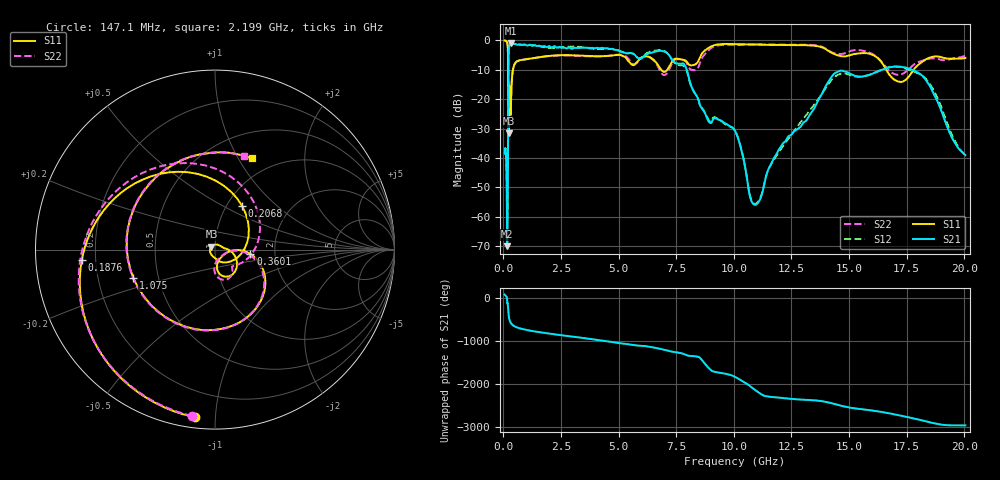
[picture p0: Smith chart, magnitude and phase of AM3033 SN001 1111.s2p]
# Hz S DB R 50
!freq MagS11 AngS11 MagS21 AngS21 MagS12 AngS12 MagS22 AngS22
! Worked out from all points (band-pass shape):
!   1601 points, 50 MHz to 20.05 GHz, reference 50 ohm
!   highest |S21| = -0.93 dB at 335.3 MHz (marker M1); lowest = -69.9 dB at 162.1 MHz (marker M2)
!   |S21| within 3 dB of the highest: 226.9 MHz to 5.122 GHz (4.895 GHz wide, 183 % of centre); 6.555 GHz to 7.022 GHz (466.9 MHz wide, 6.88 % of centre)
!   lowest |S11| = -31.6 dB at 225.4 MHz (marker M3), VSWR 1.05, Z = 48 + j1.65 ohm
!   |S11| at or under -10 dB: 205.8 MHz to 413.2 MHz (207.4 MHz wide, 67 % of centre); 6.839 GHz to 7.113 GHz (273.3 MHz wide, 3.92 % of centre); 16.61 GHz to 17.81 GHz (1.195 GHz wide, 6.94 % of centre)
!   |S22| runs from -25.9 to -0.1 dB; largest |S21 - S12| = 0.064
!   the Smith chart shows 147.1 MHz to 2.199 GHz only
!   S11 on the Smith chart (normalised r, x): 147.1 MHz: 0.05, -0.89; 187.6 MHz: 0.15, -0.04; 206.8 MHz: 1.18, +0.62; 360.1 MHz: 1.49, -0.08; 1.075 GHz: 0.36, -0.15; 2.199 GHz: 0.78, +1.14
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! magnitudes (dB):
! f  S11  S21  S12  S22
! 50 MHz  -0.1  -38.5  -38.1  -0.1
! 135.9 MHz  -0.4  -45.9  -45.8  -0.4
! 147.1 MHz  -0.5  -53.0  -52.6  -0.6
! 162.1 MHz  -0.9  -69.9  -68.8  -0.9
! 187.6 MHz  -2.6  -50.9  -51.0  -2.7
! 206.8 MHz  -10.9  -15.7  -15.6  -8.9
! 225.4 MHz  -31.6  -4.2  -4.2  -17.3
! 252.2 MHz  -15.8  -2.0  -2.0  -15.0
! 307.6 MHz  -25.2  -1.0  -1.0  -25.9
! 335.3 MHz  -18.5  -0.9  -1.0  -18.5
! 360.1 MHz  -14.0  -1.0  -1.0  -14.0
! 369.6 MHz  -12.9  -1.0  -1.0  -12.9
! 1.005 GHz  -6.5  -1.8  -1.5  -6.4
! 1.075 GHz  -6.3  -1.7  -1.6  -6.3
! 2.199 GHz  -5.2  -2.0  -2.6  -5.3
! 2.722 GHz  -5.1  -2.8  -2.4  -5.1
! 7.402 GHz  -6.5  -7.3  -7.6  -6.9
! 9.951 GHz  -1.3  -29.7  -29.8  -1.5
! 10.93 GHz  -1.4  -55.9  -55.6  -1.4
! 14.64 GHz  -5.4  -10.3  -11.4  -4.7
! 17.92 GHz  -9.0  -10.6  -11.0  -7.7
! 20.05 GHz  -6.0  -39.0  -39.0  -5.2
